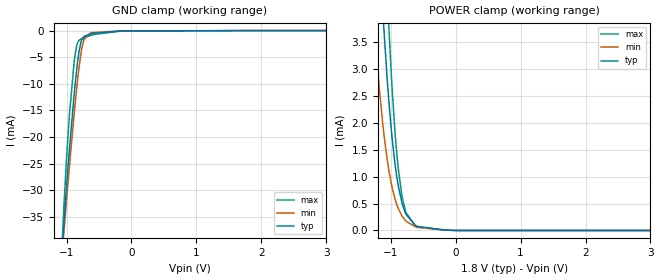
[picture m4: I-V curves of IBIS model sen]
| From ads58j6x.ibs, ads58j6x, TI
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|   sen Model
[Model]   sen
Model_type   Input
Vinl = 0.4
Vinh = 1.2
|   typ   min   max
|   (nom PVT)   (fast PVT)   (slow PVT)
|Average
C_comp   1.163e-12   1.143e-12   1.183e-12
| Where nom  PVT is Nominal Process, 1.8V, 25C
|   Fast PVT is Strong Process,  1.9V, -40C
|   Slow PVT is Weak Process,   1.7V, 85C
[Voltage Range]   1.8   1.7   1.9
|Ambient Temperature   25   85   -40
|Junction Temperature
[Temperature Range]   25   85   -40
[Power Clamp Reference]   1.8   1.7   1.9
[GND Clamp Reference]   0   0   0
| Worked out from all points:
|   GND clamp passes 1 mA (typ) near -0.71 V on its own axis
|   POWER clamp passes 1 mA (typ) near -0.91 V on its own axis
[GND Clamp]
|   Voltage   I(typ)   I(min)   I(max)
-1.8V     -254mA     -233.2mA   -272.2mA
-1.072V   -42.68mA   -43.04mA   -41.27mA
-1.057V   -39.59mA   -40.62mA   -37.3mA
-1.039V   -36.06mA   -37.76mA   -32.73mA
-958.3mV  -22.73mA   -25.98mA   -16.36mA
-882.3mV  -12.04mA   -15.69mA   -5.832mA
-848.1mV  -7.901mA   -11.46mA   -3.044mA
-806.4mV  -3.894mA   -6.889mA   -1.82mA
-732.2mV  -1.099mA   -1.716mA   -1.358mA
-630.4mV  -627.8uA   -459.5uA   -912uA
-180mV    -94uA      -76.45uA   -118.4uA
3.6V      0A         0A         0A
[POWER Clamp]
|   Voltage   I(typ)   I(min)   I(max)
-1.8V     24.81mA    16.7mA     34.5mA
-1.251V   7.152mA    3.78mA     10.93mA
-1.171V   5.168mA    2.582mA    8.058mA
-1.101V   3.674mA    1.758mA    5.797mA
-1.028V   2.398mA    1.117mA    3.77mA
-935.5mV  1.252mA    593uA      1.859mA
-884.2mV  833.5uA    410.7uA    1.157mA
-829.1mV  525.2uA    275.8uA    660.3uA
-763.2mV  297.8uA    172.6uA    327.1uA
-618.5mV  91.86uA    67.42uA    82.22uA
1.8mV     26.04nA    147nA      27.06nA
3.6V      0A         0A         0A
